PROGRAM Main
VAR
	bEnable: BOOL := TRUE;		(*enable or disable the functionblock by changing the value of this variable*)
	fbOcaDevice: FB_OcaDevice;	(*instance of the function block which represents the OCA Device*)
	fbOcaRoot: FB_OcaRoot;		(*instance of the function block which represents the OCA Object*)

	{attribute hide}	bInit: BOOL;	(*will be TRUE after the first cycle*) 

	stRole: ST_StringProperty;			(*structure which will contain the result 'Role' *)

	bLock: BOOL;						(*	Locks the object so that it can only be accessed by the lockholder. The return value indicates
											whether the operation succeeded (the OcaStatus is shown by the value of eState).	
											Lock / Unlock could be done easily to test the functionality as shown here: 
											https://infosys.beckhoff.de/english.php?content=../content/1033/tc3_userinterface/html/write_values.htm&id=4588647580592689371
										*)
	_bLock: BOOL;						(*only used to recognize changes*)
	stObjectLocked: ST_BooleanProperty;	(*structure which will contain the result 'Object locked' *)
END_VAR

A_Init();		(*enter IP Address and other parameters of the device in this Action*)  
A_Operation();

ACTION A_Init:
IF NOT bInit THEN
	bInit := TRUE;

	(* ----------- Init devices -------------*)
	InitDeviceList();
	fbOcaDevice.sDeviceName := 'Amplifier_2';

	fbOcaDevice.bLocalOcaDevice := FALSE;

	
	(* ----------- Init the object (assigned to a device) -------------*)
	InitOcaObjectList();
	fbOcaRoot.__setsOcaObjectDescription(sOcaObjectDescription := 'PwrOn', pLink := fbOcaDevice.pLink); 

END_IF
END_ACTION

ACTION A_Operation:
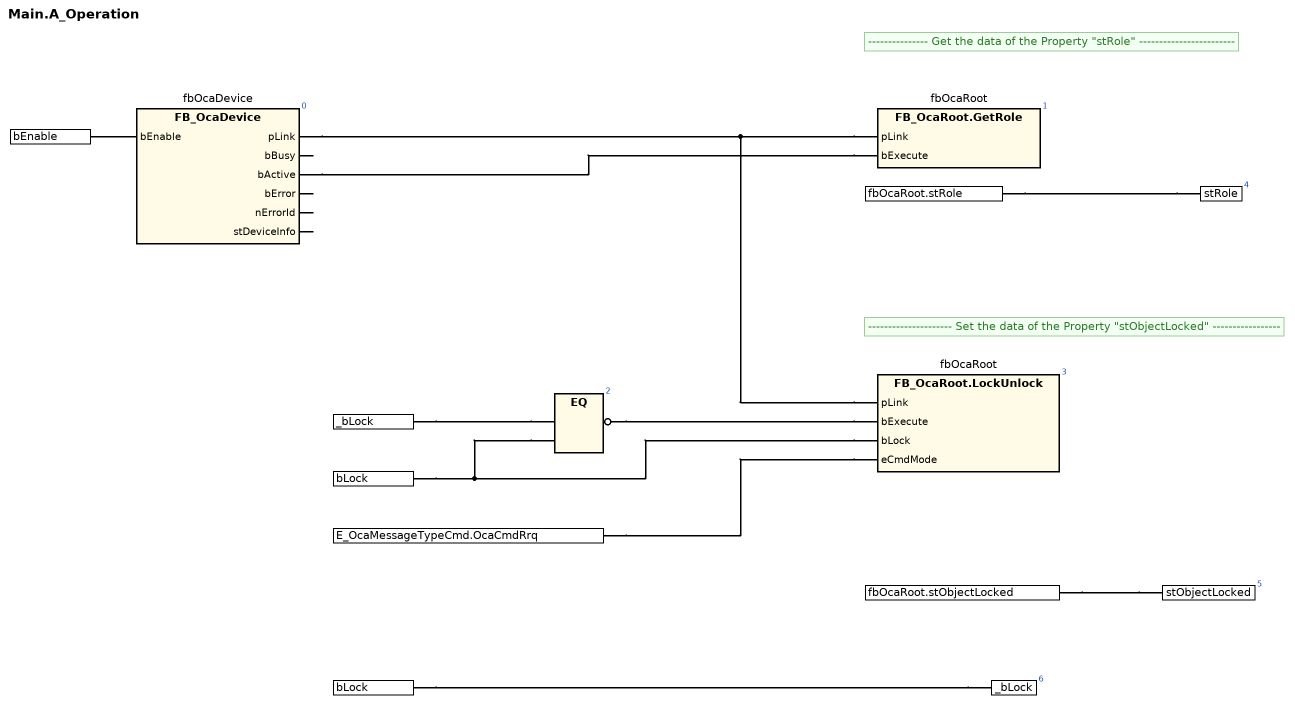
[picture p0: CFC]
fbOcaDevice(bEnable := bEnable); // FB_OcaDevice
// --------------- Get the data of the Property "stRole" ------------------------
fbOcaRoot.GetRole(pLink := fbOcaDevice.pLink, bExecute := fbOcaDevice.bActive);
// --------------------- Set the data of the Property "stObjectLocked" -----------------
fbOcaRoot.LockUnlock(pLink := fbOcaDevice.pLink, bExecute := NOT (_bLock = bLock), bLock := bLock, eCmdMode := E_OcaMessageTypeCmd.OcaCmdRrq);
stRole := fbOcaRoot.stRole;
stObjectLocked := fbOcaRoot.stObjectLocked;
_bLock := bLock;
END_ACTION

(* set parameters of the device *)
METHOD InitDeviceList
VAR
	i: INT  (0..(GVL_AES70.MAX_DEVICES - 1)) := 0;	//variable only used to count during initialization  
END_VAR

GVL_AES70.aOcaDevices[i].ipAddr := '169.254.40.175';		// the ip addres of the first device
GVL_AES70.aOcaDevices[i].ipPort := 30013;				// the port of the first device
GVL_AES70.aOcaDevices[i].sDeviceName := 'Amplifier_1';	// the unique name of the first device 

i:=i+1;
GVL_AES70.aOcaDevices[i].ipAddr := '169.254.1.7';	// the ip addres of the second device
GVL_AES70.aOcaDevices[i].ipPort := 30013;				// the port of the second device
GVL_AES70.aOcaDevices[i].sDeviceName := 'Amplifier_2';	// the unique name of the second device 

i:=i+1;
GVL_AES70.aOcaDevices[i].ipAddr := '169.254.163.144';	// the ip addres of the third device
GVL_AES70.aOcaDevices[i].ipPort := 42502;				// the port of the third device
GVL_AES70.aOcaDevices[i].sDeviceName := 'Amplifier_3';	// the unique name of the third device
END_METHOD

(* set parameters of the objects *)
METHOD InitOcaObjectList
VAR
	i: 	UINT  (0..(GVL_AES70.MAX_DEVICES - 1)) := 0;				//variable only used to count during initialization
	ii: UINT  (0..(GVL_AES70.MAX_OBJECTS_PER_DEVICE - 1)) := 0;	//variable only used to count during initialization  
END_VAR
(*Objects used by the first device*)
GVL_AES70.aOcaDevices[i].aOcaObjectList[ii].nOcaObjectNr := 16#10000100;
GVL_AES70.aOcaDevices[i].aOcaObjectList[ii].nOwnerNr := 16#10001FE;
GVL_AES70.aOcaDevices[i].aOcaObjectList[ii].sDescription := 'PwrOn';

(*Copy all above defined Oca Objects to the other devices*)
i:= i+1;
GVL_AES70.aOcaDevices[i].aOcaObjectList := GVL_AES70.aOcaDevices[0].aOcaObjectList;
i:= i+1;
GVL_AES70.aOcaDevices[i].aOcaObjectList := GVL_AES70.aOcaDevices[0].aOcaObjectList;
END_METHOD

END_PROGRAM
